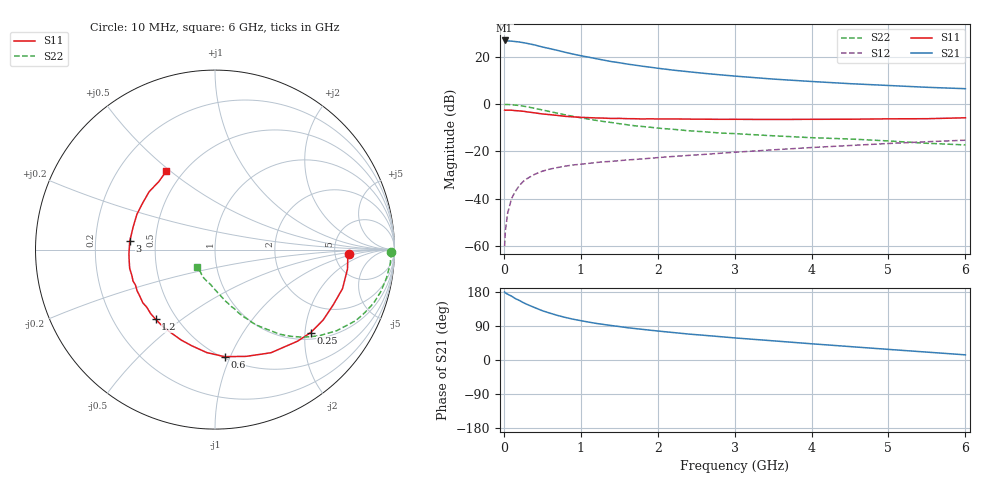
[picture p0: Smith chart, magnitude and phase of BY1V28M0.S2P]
! SIEMENS Small Signal Semiconductors
! BFY420
! Si NPN RF SIEGET Grounded Emitter Transistor in MICRO-X
! VCE = 1.25 V  IC = 8 mA
! Common Emitter S-Parameters:  October  1996
# GHz  S  MA  R  50
!  f  S11  S21  S12  S22
! GHz  MAG  ANG  MAG  ANG  MAG  ANG  MAG  ANG
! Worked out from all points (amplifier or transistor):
!   36 points, 10 MHz to 6 GHz, reference 50 ohm
!   highest |S21| = 26.9 dB at 10 MHz (marker M1)
!   |S21| within 3 dB of that: start of sweep to 535.2 MHz
!   unconditionally stable (mu >= 1): 2.621 GHz to end of sweep
!   at 250 MHz: K = 0.14, MSG = 29.3 dB, |S12| = -32.7 dB
!   at 1.4 GHz: K = 0.70, MSG = 21.1 dB, |S12| = -24.2 dB
!   at 6 GHz: K = 1.12, MAG = 8.7 dB, |S12| = -15.2 dB
!   S11 on the Smith chart (normalised r, x): 10 MHz: 6.86, -0.77; 250 MHz: 1.16, -2.14; 600 MHz: 0.51, -0.95; 1.2 GHz: 0.39, -0.40; 3 GHz: 0.35, +0.04; 6 GHz: 0.41, +0.48
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0.01  0.7483 -1.9  22.07 179.5  0.001 97.1  0.9797 -0.8
0.02  0.7412 -3.6  21.94 177.1  0.0021 78.6  0.9819 -1.7
0.1  0.7431 -17.0  21.39 168.6  0.0101 81.1  0.9684 -9.5
0.15  0.7272 -25.0  20.91 162.0  0.0144 77.0  0.9529 -14.2
0.2  0.719 -33.1  20.5 157.3  0.0189 74.3  0.9336 -18.5
0.25  0.7058 -40.9  19.86 151.7  0.0231 71.3  0.9063 -22.7
0.3  0.6869 -48.0  19.19 146.8  0.0266 67.6  0.8792 -26.7
0.4  0.6538 -61.5  17.75 138.4  0.0329 62.1  0.8147 -33.7
0.5  0.6198 -73.7  16.09 130.1  0.0383 56.9  0.7523 -39.7
0.6  0.5988 -84.9  14.8 123.6  0.0425 54.0  0.6939 -44.7
0.7  0.5755 -94.6  13.59 117.5  0.0458 50.8  0.641 -48.9
0.8  0.5514 -103.5  12.39 112.3  0.049 48.2  0.5921 -52.7
0.9  0.538 -110.5  11.38 107.7  0.0519 47.1  0.5498 -55.4
1.1  0.518 -124.2  9.813 100.1  0.056 44.8  0.4823 -61.0
1.2  0.5101 -130.4  9.102 96.6  0.0584 44.0  0.4534 -63.2
1.6  0.4924 -148.7  7.019 85.4  0.0661 42.2  0.3668 -70.3
2.2  0.4867 -167.6  5.219 72.5  0.0784 41.1  0.2938 -78.4
3  0.4774 174.5  3.905 58.3  0.0962 39.2  0.238 -86.8
3.5  0.4731 164.4  3.376 50.6  0.1082 37.2  0.2143 -92.2
4.5  0.4795 147.0  2.7 35.4  0.1336 31.2  0.1831 -103.8
5.5  0.4915 129.6  2.264 20.8  0.1605 23.7  0.1488 -123.2
6  0.5142 121.9  2.115 13.6  0.1729 19.5  0.1373 -136.5
